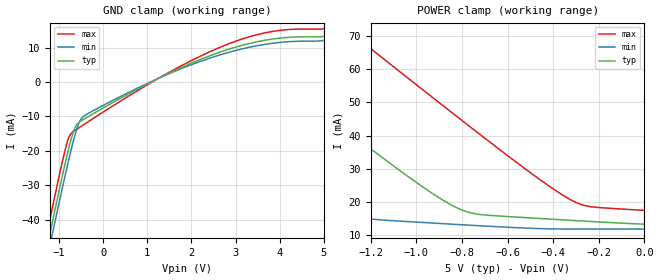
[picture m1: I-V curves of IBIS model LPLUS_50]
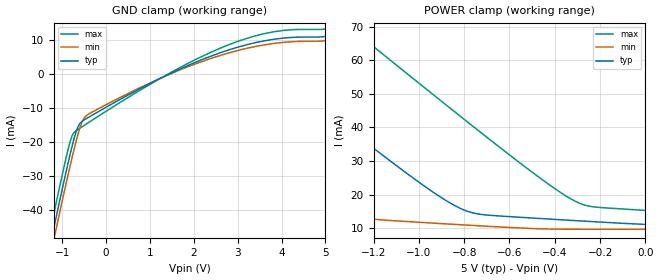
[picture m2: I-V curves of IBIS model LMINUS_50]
| TEXAS INSTRUMENTS INCORPORATED
| Standard Linear and Logic Group
| IBIS Model of UCC5672
| Multimod SCSI 9 Line Terminator
| This file contains package information for the following:
|  TSSOP 28-pin (pwp) package as [Component] UCC5672_pwp
| This device can be powered at the following Vccs:
|  5 volt Vcc
| This file provides unique models under the [Model Selector] for each Vcc.
| For operation at a specific Vcc, select the appropriate model after each
| [Model Selector] keyword.
[IBIS Ver]   3.2
[Comment char]  |_char
[File Name]   ucc5672_pwp_lvd.ibs
[File Rev]   1.0 |
[Date]   March 28, 2004
[Source]   Data created from TI-SPICE simulations at TI-SLL.
[Notes]   The following is an IBIS list for the UCC5672.
   Please contact sllibis@ti.com with questions and
   comments concerning SLL IBIS models.
[Disclaimer] Property of Texas Instruments Incorporated.  Unauthorized
   reproduction and/or distribution is strictly prohibited.
   This product is protected under copyright law.
   Created  2004, (C) Copyright  2004, Texas Instruments
   Incorporated, All Rights Reserved
   UNLESS THERE IS A SIGNED, WRITTEN AGREEMENT TO THE
   CONTRARY, TEXAS INSTRUMENTS (TI) IS PROVIDING THE IBIS
   MODELS  AND WITHOUT ANY WARRANTY, EXPRESSED OR
   IMPLIED.  TI assumes no liability for:
   1) the accuracy of the IBIS models provided to your
   company;
   2) the proper functioning of these IBIS Models in your
   design or for any resulting applications; or
   3) infringement of patents, copyrights or intellectual
   property rights resulting from your use of these IBIS
   models.
   TI provides IBIS Models as a service to our customers.
   You and your company shall not distribute, sell or give
   these models to anyone else without prior written
   permission from TI.
   TI reserves the right to make changes to our products or
   to discontinue any semiconductor product or service
   without notice, and advises our customers to obtain the
   latest version of relevant information to verify, before
   placing orders, that the information being relied on is
   current.
   Please be aware that your receipt and use of the IBIS
   information provided shall serve as acceptance of these
   terms and conditions.  If you do not accept these terms,
   you should return or destroy the IBIS models and any
   other accompanying information immediately.
| Component UCC5672_pwp 28-pin QSOP
[Component]   UCC5672_pwp
[Manufacturer]   Texas Instruments, Inc.
[Package]
|   typ   min   max
R_pkg   1.0786E-01	7.5230E-02	1.4375E-01
L_pkg   1.4406E+00	9.3821E-01	1.9964E+00
C_pkg   9.6530E-02	6.5460E-02	1.5751E-01
[Pin] signal   model  R_pin   L_pin   C_pin
1	REG 	 POWER 	0.14088	1.95052	0.1359
2	L1PLUS 	 LPLUS 	0.1386	1.9143	0.13637
3	L1MINUS  LMINUS 0.14209	1.96969	0.12232
4	L2PLUS 	 LPLUS 	0.12872	1.75932	0.11211
5	L2MINUS  LMINUS 0.10092	1.32607	0.09259
6	HSGND 	 GND 	0.08255	1.04595	0.07191
7	L3PLUS 	 LPLUS 	0.09174	1.18562	0.07833
8	L3MINUS  LMINUS 0.07919	0.99619	0.07156
9	L4PLUS 	 LPLUS 	0.07523	0.93821	0.06807
10	L4MINUS  LMINUS 0.07704	0.967	0.06989
11	L5PLUS 	 LPLUS 	0.09231	1.20027	0.08294
12	L5MINUS  LMINUS 0.1146	1.54626	0.09787
13	DISCNCT  POWER 	0.13992	1.94528	0.11951
14	GND 	 GND 	0.1387	1.92611	0.15751
15	NC 	 NC 	0.13621	1.88698	0.11333
16	DIFFSENS POWER 	0.13733	1.90453	0.11733
17	DIFFB 	 POWER 	0.11845	1.6065	0.10336
18	L6PLUS 	 LPLUS 	0.09319	1.2138	0.0847
19	L6MINUS  LMINUS 0.07748	0.97361	0.07031
20	L7PLUS 	 LPLUS 	0.07531	0.93952	0.06793
21	L7MINUS  LMINUS 0.07894	0.9924	0.06806
22	HSGND 	 GND 	0.07561	0.94343	0.06546
23	L8PLUS 	 LPLUS 	0.0797	1.00317	0.07194
24	L8MINUS  LMINUS 0.09653	1.25854	0.08436
25	L9PLUS 	 LPLUS 	0.12244	1.66127	0.10118
26	L9MINUS  LMINUS 0.14375	1.99637	0.12231
27	TRMPWR 	 POWER 	0.14098	1.95214	0.12264
28	TRMPWR 	 POWER 	0.10155	1.33452	0.09306
[Diff Pin]  inv_pin   vdiff   tdelay_typ
2   3   NA   NA
4   5   NA   NA
7   8   NA   NA
9   10   NA   NA
11   12   NA   NA
18   19   NA   NA
20   21   NA   NA
23   24   NA   NA
25   26   NA   NA
| Model LPLUS
[Model Selector]   LPLUS
LPLUS_50   5 volt Vcc
| Model LMINUS
[Model Selector]   LMINUS
LMINUS_50   5 volt Vcc
| Models and submodels in the file (2): LPLUS_50 (Input), LMINUS_50 (Input)
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[Model]   LPLUS_50
Model_type  Input
Vinl=0.8
Vinh=2.0
| variable   typ   min   max
C_comp   0.58pF   0.32pF   0.96pF
[Temperature Range]   40   100   -40
| Ambient temperature   25   85   -40
[Voltage range]   5   5   5
[GND Clamp]
| LPLUS_50
|   Voltage   I(typ)   I(min)   I(max)
-5V       -283.8mA   -285.2mA   -282.8mA
-1.36V    -53.33mA   -56.65mA   -49.38mA
-1.235V   -45.7mA    -49.09mA   -41.63mA
-1.16V    -41.15mA   -44.59mA   -37.02mA
-780mV    -19.22mA   -22.57mA   -16.11mA
-630mV    -12.98mA   -14.96mA   -13.98mA
-530mV    -11.53mA   -11.36mA   -13.13mA
-420mV    -10.66mA   -9.729mA   -12.2mA
1.28V     1.26mA     1.241mA    1.29mA
2.79V     9.33mA     8.45mA     10.85mA
3.835V    12.52mA    11.28mA    14.73mA
5V        13.35mA    12.13mA    15.56mA
[POWER Clamp]
| LPLUS_50
|   Voltage   I(typ)   I(min)   I(max)
-5V       243.8mA    213.5mA    275.7mA
-2.42V    101.7mA    72.17mA    133.1mA
-1.895V   73.12mA    44.13mA    104.2mA
-1.825V   69.33mA    40.47mA    100.3mA
-1.485V   51.03mA    23.46mA    81.71mA
-1.3V     41.22mA    16.33mA    71.61mA
-960mV    24mA       13.82mA    53.16mA
-780mV    17.13mA    13.11mA    43.5mA
-465mV    15.1mA     12.04mA    27.12mA
-310mV    14.47mA    11.92mA    20.24mA
-230mV    14.16mA    11.91mA    18.57mA
-84.45fV  13.35mA    11.91mA    17.5mA
[Model]   LMINUS_50
Model_type  Input
Vinl=0.8
Vinh=2.0
| variable   typ   min   max
C_comp   0.58pF   0.31pF   0.97pF
[Temperature Range]   40   100   -40
| Ambient temperature   25   85   -40
[Voltage range]   5   5   5
[GND Clamp]
| LMINUS_50
|   Voltage   I(typ)   I(min)   I(max)
-5V       -286mA     -287.3mA   -284.9mA
-1.36V    -55.47mA   -58.79mA   -51.52mA
-1.235V   -47.84mA   -51.23mA   -43.77mA
-1.16V    -43.29mA   -46.73mA   -39.16mA
-790mV    -21.89mA   -25.25mA   -18.59mA
-630mV    -15.12mA   -17.1mA    -16.12mA
-530mV    -13.67mA   -13.5mA    -15.27mA
-420mV    -12.8mA    -11.87mA   -14.34mA
1.28V     -880.2uA   -898.6uA   -850.3uA
2.79V     7.19mA     6.31mA     8.712mA
3.835V    10.38mA    9.143mA    12.59mA
5V        11.21mA    9.988mA    13.42mA
[POWER Clamp]
| LMINUS_50
|   Voltage   I(typ)   I(min)   I(max)
-5V       241.7mA    211.4mA    273.6mA
-2.42V    99.59mA    70.03mA    130.9mA
-2.315V   93.85mA    64.37mA    125.2mA
-1.895V   70.98mA    41.99mA    102.1mA
-1.825V   67.19mA    38.33mA    98.2mA
-1.465V   47.82mA    20.4mA     78.48mA
-1.29V    38.55mA    13.96mA    68.92mA
-935mV    20.7mA     11.58mA    49.67mA
-780mV    14.99mA    10.97mA    41.36mA
-310mV    12.33mA    9.775mA    18.1mA
-230mV    12.02mA    9.773mA    16.43mA
-84.45fV  11.21mA    9.765mA    15.37mA
